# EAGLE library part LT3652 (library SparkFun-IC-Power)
LT3652 MPPT Solar Charge Controller(IC-11822) 5V-32V smart charger for batteries up to 14.4V
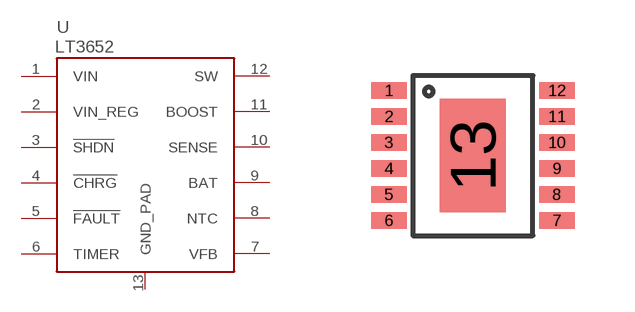
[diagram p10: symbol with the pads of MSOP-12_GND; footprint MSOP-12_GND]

Designator prefix U

## LT3652 (VALUE: LT3652)  [MSOP-12_GND]
1  VIN
2  VIN_REG
3  !SHDN
4  !CHRG
5  !FAULT
6  TIMER
7  VFB
8  NTC
9  BAT
10  SENSE
11  BOOST
12  SW
13  GND_PAD

## Footprint MSOP-12_GND (pad centres in mm)
smd 0.889 x 0.42: 1 -2.1,1.625; 2 -2.1,0.975; 3 -2.1,0.325; 4 -2.1,-0.325; 5 -2.1,-0.975; 6 -2.1,-1.625; 7 2.1,-1.625; 8 2.1,-0.975; 9 2.1,-0.325; 10 2.1,0.325; 11 2.1,0.975; 12 2.1,1.625
smd 1.651 x 2.845: 13 0,0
